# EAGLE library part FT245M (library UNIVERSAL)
FT 245 mini modul SMD
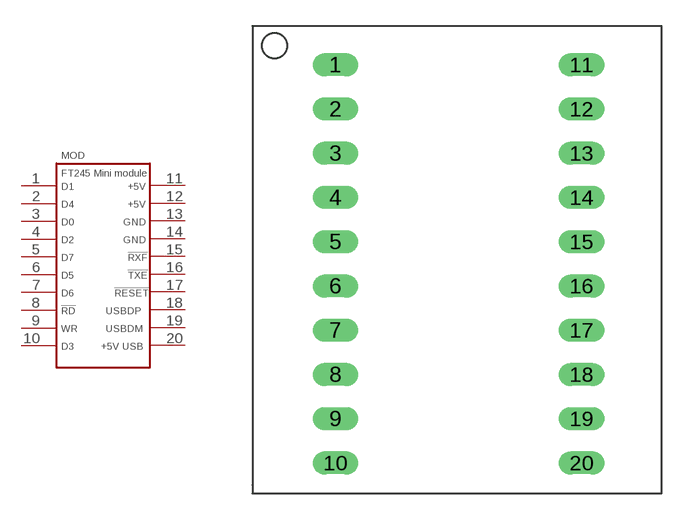
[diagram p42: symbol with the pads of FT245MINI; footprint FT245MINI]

Designator prefix MOD

## FT245M  [FT245MINI]
1  1
2  2
3  3
4  4
5  5
6  6
7  7
8  8  in
9  9  in
10  10
11  11  pwr
12  12  pwr
13  13  pwr
14  14  pwr
15  15  out
16  16  out
17  17  in
18  18
19  19
20  20  in

## Footprint FT245MINI (pad centres in mm)
drill 0.8 long: 1 0,22.86; 2 0,20.32; 3 0,17.78; 4 0,15.24; 5 0,12.7; 6 0,10.16; 7 0,7.62; 8 0,5.08; 9 0,2.54; 10 0,0; 11 14.129,22.86; 12 14.129,20.32; 13 14.129,17.78; 14 14.129,15.24; 15 14.129,12.7; 16 14.129,10.16; 17 14.129,7.62; 18 14.129,5.08; 19 14.129,2.54; 20 14.129,0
